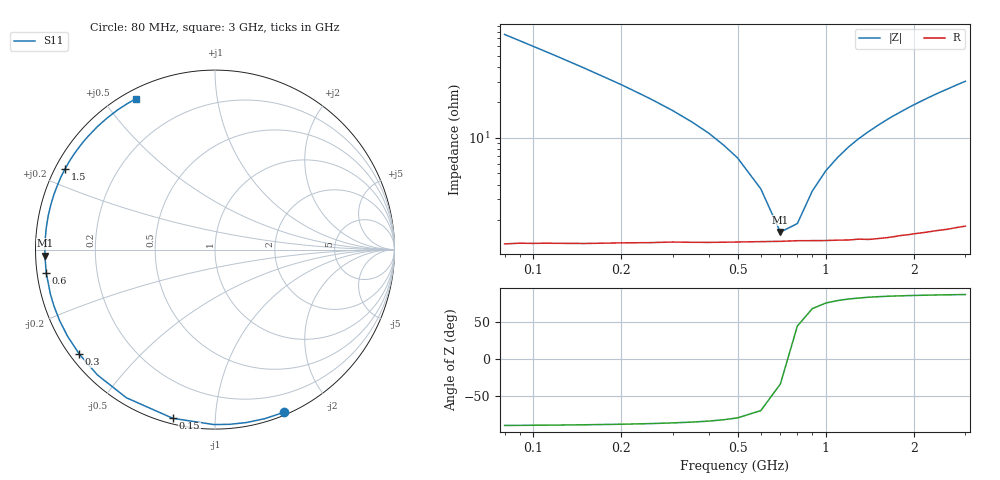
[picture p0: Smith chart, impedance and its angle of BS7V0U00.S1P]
! SIEMENS Small Signal Semiconductors
! BB640
! Si Tuning Diode in SOD323
! VR = 7 V
! S-Parameters:  July  1993
# GHz  S  MA  R  50
!  f  S11
! GHz  MAG  ANG
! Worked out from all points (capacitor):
!   33 points, 80 MHz to 3 GHz, reference 50 ohm
!   read as one part to ground: C = 26 pF near 80 MHz
!   lowest |Z| = 1.58 ohm at 700 MHz (marker M1)
!   series resonance near 740 MHz, so ESL is about 1.8 nH
!   S11 on the Smith chart (normalised r, x): 80 MHz: 0.03, -1.51; 150 MHz: 0.03, -0.78; 300 MHz: 0.03, -0.34; 600 MHz: 0.03, -0.07; 1.5 GHz: 0.03, +0.25; 3 GHz: 0.04, +0.60
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0.08  0.9848 -67.0
0.09  0.9819 -73.5
0.1  0.9794 -79.6
0.11  0.9769 -85.2
0.12  0.9747 -90.4
0.15  0.969 -104.0
0.2  0.9619 -120.9
0.25  0.9575 -133.2
0.3  0.9543 -142.4
0.35  0.9528 -149.7
0.4  0.9517 -155.6
0.45  0.9507 -160.7
0.5  0.95 -164.9
0.6  0.949 -172.1
0.7  0.9485 -178.0
0.8  0.9479 177.0
0.9  0.948 172.5
1  0.9482 168.4
1.2  0.9485 161.1
1.3  0.9482 157.8
1.5  0.9489 151.7
1.6  0.9488 148.8
1.8  0.948 143.4
2  0.9479 138.3
2.2  0.948 133.6
2.4  0.9481 129.2
2.8  0.9487 121.3
3  0.9492 117.7
